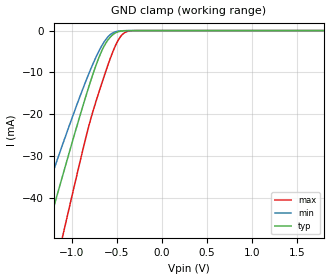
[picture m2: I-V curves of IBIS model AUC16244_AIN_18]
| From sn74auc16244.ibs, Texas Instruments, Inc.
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[Model]   AUC16244_AIN_18
Model_type  Input
Vinl=0.5775
Vinh=1.2675
| variable   typ   min   max
C_comp   3.28pF   2.59pF   3.84pF
[Temperature Range]   40   100   -40
| Ambient temperature   25   85   -40
[Voltage range]   1.8   1.65   1.95
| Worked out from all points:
|   GND clamp passes 1 mA (typ) near -0.54 V on its own axis
[GND Clamp]
| AUC16244_AIN_18
|   Voltage   I(typ)   I(min)   I(max)
-3.6V     -231.9mA   -193.8mA   -279.4mA
-1.43V    -60.24mA   -48.06mA   -80.04mA
-1.295V   -49.73mA   -39.44mA   -67.46mA
-1.255V   -46.64mA   -36.91mA   -63.73mA
-1.095V   -34.38mA   -26.96mA   -48.81mA
-1.05V    -30.97mA   -24.22mA   -44.62mA
-815mV    -13.9mA    -10.68mA   -23.37mA
-680mV    -5.605mA   -4.247mA   -13.65mA
-560mV    -1.339mA   -800.2uA   -6.09mA
-485mV    -307.4uA   -149.3uA   -2.421mA
-420mV    -59.16uA   -28.47uA   -643uA
1.8V      219.3pA    320.6pA    252.3pA
